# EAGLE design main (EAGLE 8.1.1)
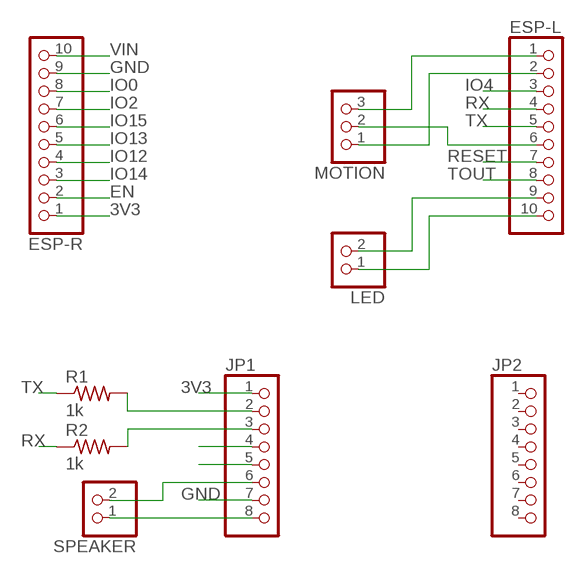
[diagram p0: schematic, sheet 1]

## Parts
ESP-L  PINHD-1X10  [1X10]
ESP-R  PINHD-1X10  [1X10]
JP1  PINHD-1X8  [1X08]
JP2  PINHD-1X8  [1X08]
LED  PINHD-1X2  [1X02]
MOTION  PINHD-1X3  [1X03]
R1  1k  RES-US1206FAB  [R1206FAB]
R2  1k  RES-US1206FAB  [R1206FAB]
SPEAKER  PINHD-1X2  [1X02]

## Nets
3V3: ESP-R.1 JP1.1
EN: ESP-R.2
GND: ESP-R.9 JP1.7
IO0: ESP-R.8
IO2: ESP-R.7
IO4: ESP-L.3
IO12: ESP-R.4
IO13: ESP-R.5
IO14: ESP-R.3
IO15: ESP-R.6
N$1: ESP-L.1 MOTION.3
N$2: ESP-L.2 MOTION.1
N$3: ESP-L.6 MOTION.2
N$4: JP1.6 SPEAKER.2
N$5: ESP-L.10 LED.1
N$6: ESP-L.9 LED.2
N$7: JP1.8 SPEAKER.1
N$8: JP1.2 R1.2
N$9: JP1.4
N$10: JP1.5
N$11: JP1.3 R2.2
RESET: ESP-L.7
RX: ESP-L.4 R2.1
TOUT: ESP-L.8
TX: ESP-L.5 R1.1
VIN: ESP-R.10
Unconnected: JP2.1 JP2.2 JP2.3 JP2.4 JP2.5 JP2.6 JP2.7 JP2.8

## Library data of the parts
ESP-L ESP-R = pinhead:PINHD-1X10: PIN HEADER
JP1 JP2 = pinhead:PINHD-1X8: PIN HEADER
LED SPEAKER = pinhead:PINHD-1X2: PIN HEADER
MOTION = pinhead:PINHD-1X3: PIN HEADER
R1 R2 = fab:RES-US: Resistor (US Symbol)

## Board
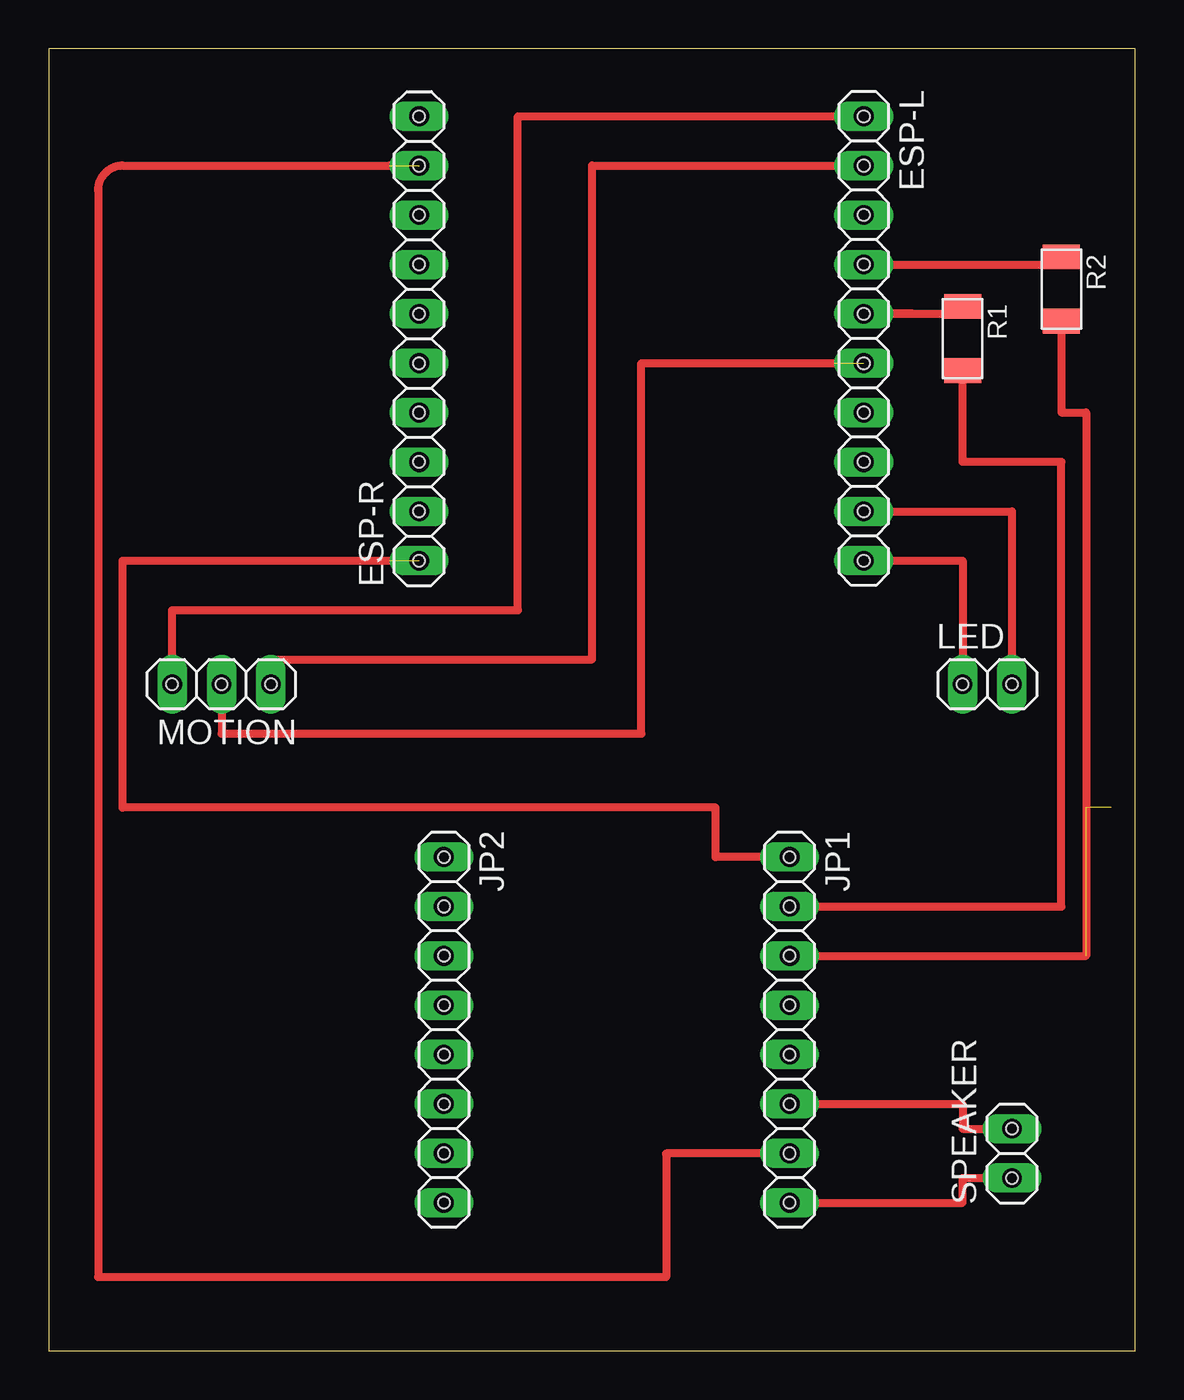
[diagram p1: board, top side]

Size 55.86 x 66.98 mm. Coordinates in mm from the lower left corner, seen from the top.
Outline: 0,0 55.86,0 55.86,66.98 0,66.98 0,0
Copper layers (1*16): Top 0.035mm / dielectric 1.5mm / Bottom 0.035mm
Design rules "default *": minimum track width 10mil, minimum drill 24mil, track to track 0.4mm, track to pad 0.4mm, pad to pad 0.4mm, via to via 0.4mm, smd to smd 0.4mm, copper to edge 40mil, drill to drill 8mil, minimum pad ring 10mil, minimum via ring 8mil, stop-mask expansion 4mil, vias tented up to drill 0mil, thermal gap 10mil
Holes 0.6 mm at 6.35,34.29 8.89,34.29 11.43,34.29 19.05,40.64 19.05,43.18 19.05,45.72 19.05,48.26 19.05,50.8 19.05,53.34 19.05,55.88 19.05,58.42 19.05,60.96 19.05,63.5 41.91,63.5 41.91,60.96 41.91,58.42 41.91,55.88 41.91,53.34 41.91,50.8 41.91,48.26 41.91,45.72 41.91,43.18 41.91,40.64 46.99,34.29 49.53,34.29 20.32,25.4 20.32,22.86 20.32,20.32 20.32,17.78 20.32,15.24 20.32,12.7 20.32,10.16 20.32,7.62 38.1,15.24 38.1,12.7 38.1,10.16 38.1,7.62 38.1,25.4 38.1,22.86 38.1,20.32 38.1,17.78 49.53,11.43 49.53,8.89

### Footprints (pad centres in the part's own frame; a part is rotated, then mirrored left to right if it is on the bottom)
1X10 = drill 1.016 long: 1 -11.43,0; 2 -8.89,0; 3 -6.35,0; 4 -3.81,0; 5 -1.27,0; 6 1.27,0; 7 3.81,0; 8 6.35,0; 9 8.89,0; 10 11.43,0
1X08 = drill 1.016 long: 1 -8.89,0; 2 -6.35,0; 3 -3.81,0; 4 -1.27,0; 5 1.27,0; 6 3.81,0; 7 6.35,0; 8 8.89,0
1X02 = drill 1.016 long: 1 -1.27,0; 2 1.27,0
1X03 = drill 1.016 long: 1 -2.54,0; 2 0,0; 3 2.54,0
R1206FAB = smd 1.27 x 1.905: 1 -1.651,0; 2 1.651,0

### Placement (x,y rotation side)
ESP-L  41.91,52.07 270 top
ESP-R  19.05,52.07 90 top
JP1  38.1,16.51 270 top
JP2  20.32,16.51 270 top
LED  48.26,34.29 0 top
MOTION  8.89,34.29 180 top
R1  46.99,52.07 270 top
R2  52.07,54.61 270 top
SPEAKER  49.53,10.16 90 top

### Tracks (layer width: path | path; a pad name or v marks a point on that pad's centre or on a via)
3V3  (1 unrouted)
  Top 0.406: 17.53,40.64 3.81,40.64 3.81,27.94 34.29,27.94 34.29,25.4 JP1.1
GND  (1 unrouted)
  Top 0.406: 17.53,60.96 3.81,60.96 arc90 2.54,59.69 2.54,3.81 31.75,3.81 31.75,10.16 JP1.7
N$1
  Top 0.406: MOTION.3 6.35,38.1 24.13,38.1 24.13,63.5 ESP-L.1
N$2
  Top 0.406: MOTION.1 11.43,35.56 27.94,35.56 27.94,60.96 ESP-L.2 43.18,60.96
N$3  (1 unrouted)
  Top 0.406: MOTION.2 8.89,31.75 30.48,31.75 30.48,50.8 40.39,50.8
N$4
  Top 0.406: SPEAKER.2 46.99,11.43 46.99,12.7 JP1.6
N$5
  Top 0.406: ESP-L.10 46.99,40.64 LED.1
N$6
  Top 0.406: ESP-L.9 49.53,43.18 LED.2
N$7
  Top 0.406: JP1.8 46.99,7.62 46.99,8.89 SPEAKER.1
N$8
  Top 0.406: JP1.2 52.07,22.86 52.07,45.72 46.99,45.72 R1.2
N$11  (2 unrouted)
  Top 0.406: JP1.3 53.34,20.32 53.34,48.26 52.07,48.26 R2.2 52.07,53.34
RX
  Top 0.406: ESP-L.4 52.07,55.88 R2.1
TX
  Top 0.406: R1.1 46.99,53.34 44.45,53.34 | 44.45,53.34 43.43,53.34 | ESP-L.5 44.45,53.34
